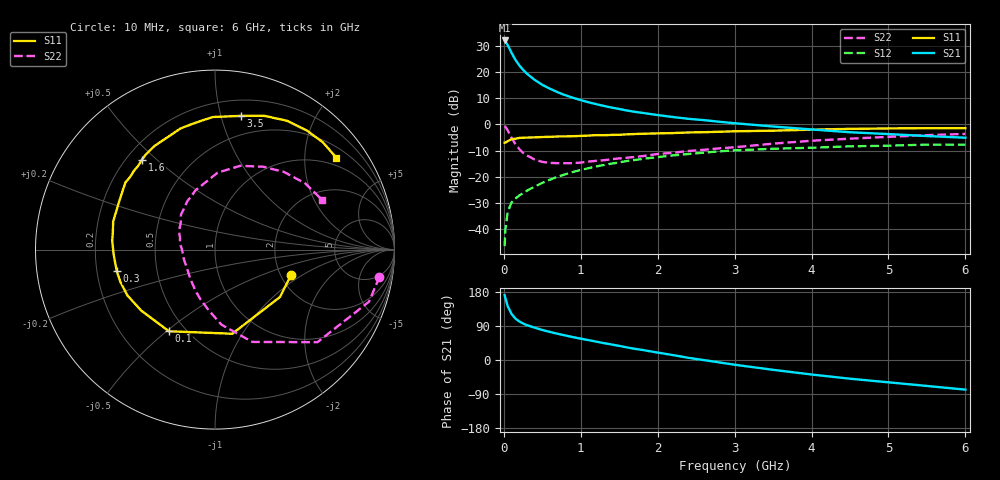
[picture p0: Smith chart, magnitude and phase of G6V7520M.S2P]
! SIEMENS Small Signal Semiconductors
! BFG193
! Si NPN RF Bipolar Junction Transistor in SOT223
! VCE = 0.75 V  IC = 20 mA
! Common Emitter S-Parameters:  August  1996
# GHz  S  MA  R  50
!  f  S11  S21  S12  S22
! GHz  MAG  ANG  MAG  ANG  MAG  ANG  MAG  ANG
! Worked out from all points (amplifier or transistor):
!   36 points, 10 MHz to 6 GHz, reference 50 ohm
!   highest |S21| = 32.1 dB at 10 MHz (marker M1)
!   |S21| within 3 dB of that: start of sweep to 71.35 MHz
!   unconditionally stable (mu >= 1): 561.5 MHz to 4.016 GHz
!   at 250 MHz: K = 0.77, MSG = 23.6 dB, |S12| = -26.3 dB
!   at 1.4 GHz: K = 1.08, MAG = 9.0 dB, |S12| = -15.0 dB
!   at 6 GHz: K = 0.98, MSG = 1.3 dB, |S12| = -7.7 dB
!   S11 on the Smith chart (normalised r, x): 10 MHz: 2.28, -0.80; 100 MHz: 0.41, -0.51; 300 MHz: 0.28, -0.10; 1.6 GHz: 0.26, +0.45; 3.5 GHz: 0.33, +1.16; 6 GHz: 0.77, +2.79
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0.01  0.447 -18.4  40.31 171.2  0.0047 84.4  0.9289 -9.4
0.02  0.4482 -36.1  39.02 163.5  0.0098 78.3  0.9059 -18.7
0.05  0.4786 -78.4  33.03 142.1  0.0211 63.4  0.7692 -42.1
0.1  0.5222 -119.4  23.45 121.8  0.0322 53.5  0.5548 -68.0
0.15  0.5333 -140.4  17.21 109.3  0.0381 50.5  0.4198 -85.1
0.2  0.5508 -152.4  13.55 101.9  0.0436 50.7  0.3394 -96.0
0.25  0.557 -161.1  11.05 96.3  0.0486 51.7  0.2861 -106.9
0.3  0.5602 -167.7  9.34 92.0  0.054 53.1  0.2546 -115.0
0.4  0.5651 -177.0  7.12 85.3  0.0648 54.3  0.2137 -129.9
0.5  0.5744 175.3  5.717 79.2  0.0762 54.8  0.1921 -142.1
0.6  0.5783 169.6  4.797 74.0  0.0879 55.2  0.1837 -151.8
0.7  0.5888 164.5  4.13 69.1  0.1 54.5  0.1817 -160.6
0.8  0.5896 159.5  3.61 64.7  0.1113 53.0  0.1811 -169.2
1.1  0.6119 146.9  2.651 52.4  0.1456 48.6  0.1948 172.1
1.3  0.6223 139.5  2.257 44.5  0.1677 44.7  0.2069 160.6
1.6  0.6458 129.0  1.844 33.3  0.1995 38.0  0.231 148.6
2.2  0.6836 111.3  1.384 12.9  0.2555 24.0  0.2868 127.2
2.8  0.7239 95.4  1.124 -6.4  0.3056 9.7  0.3486 108.0
3.5  0.7588 79.1  0.912 -25.9  0.3421 -7.8  0.4288 88.1
4.5  0.8224 60.8  0.709 -49.4  0.3809 -26.9  0.5339 59.9
5.5  0.8476 44.8  0.6 -68.5  0.4116 -48.8  0.6234 36.3
6  0.8482 37.1  0.557 -78.2  0.4106 -61.3  0.6582 24.9
